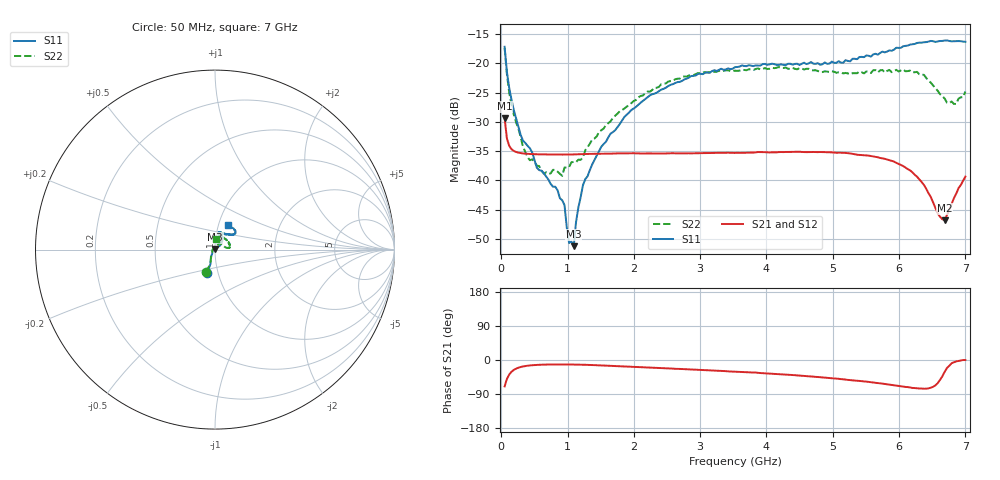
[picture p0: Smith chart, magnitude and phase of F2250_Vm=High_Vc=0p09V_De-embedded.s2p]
! Integrated Device Technology
! Corporate Headquarters
! 6024 Silver Creek Valley Road
! San Jose, CA 95138  USA
! Phone:  1-408-284-8200
! Toll Free:  1-800-223-1366
! Webpage:  http://www.idt.com/
! Timing and RF Division
! 515 Groton Road, Suite 102
! Westford, MA 01886-6024
! Device:  F2250
! Description: Voltage Variable RF Attenuator
! Frequency:  50.0 -  6000.00 MHz
! Package:  3x3 mm Thin QFN Plastic Package: 16 pin
! Ports:  2 RF, 3 DC
!  Pin  1  = GND
!  Pin  2  = NC
!  Pin  3  = RF1  = Port 1
!  Pin  4  = NC
!  Pin  5  = GND
!  Pin  6  = GND
!  Pin  7  = GND
!  Pin  8  = GND
!  Pin  9  = NC
!  Pin 10  = RF2  = Port 2
!  Pin 11  = NC
!  Pin 12  = GND
!  Pin 13  = GND
!  Pin 14  = VCNTRL
!  Pin 15  = VDD
!  Pin 16  = VMODE
! Vcntrl:  0.090 Volts
! Vmode:  +3.300 Volts
! Vdd:  +3.30  Volts
! Current:  1.245 mA
! Data:  The device was measured on a the F2250 evaluation board which has
!  individual transmission lines to the RF pins.  Data was collected
!  using a calibrated network analyzer.  The evaluation board was
!  de-embedded using a TRL calibration technique.
!  The reference plane is the edge of the package pin.
! Misc:  SN 10
!  Action Tracker AT0258
! Date Measured:  2014-11-26
! Date:  2015-10-15  MJV
! Note:
!  Integrated Device Technology supplies this data as a sample of measured
!  data at the package pin for this product.  Your particular data for this
!  product may vary.
!  Data was taken at 25 degrees C.
!  Integrated Device Technology reserves the right to change this data at anytime.
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# GHz S dB R 50
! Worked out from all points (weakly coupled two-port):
!   201 points, 50 MHz to 7 GHz, reference 50 ohm
!   highest |S21| = -29.38 dB at 50 MHz (marker M1); lowest = -46.8 dB at 6.687 GHz (marker M2)
!   lowest |S11| = -51.3 dB at 1.093 GHz (marker M3), VSWR 1.01, Z = 50 + j0.274 ohm
!   |S11| at or under -10 dB: start of sweep to end of sweep
!   |S22| runs from -39.2 to -17.4 dB; largest |S21 - S12| = 6.4e-05
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0.05  -17.18 -108.5  -29.38 -69.5  -29.38 -69.5  -17.37 -110.6
0.08475  -21.47 -107.4  -32.86 -50.1  -32.86 -50.1  -21.87 -109.0
0.15425  -26.23 -116.6  -34.68 -31.0  -34.68 -31.0  -27.10 -120.7
0.29325  -32.28 -127.5  -35.35 -18.5  -35.35 -18.4  -32.66 -133.5
0.3975  -34.11 -142.2  -35.48 -15.0  -35.48 -15.0  -36.08 -158.3
0.5365  -37.86 -154.5  -35.55 -12.9  -35.55 -12.9  -37.48 -180.0
0.64075  -38.76 -162.6  -35.58 -12.2  -35.58 -12.2  -38.88 160.6
0.91875  -43.41 156.3  -35.60 -11.8  -35.60 -11.8  -39.24 127.9
0.9535  -44.23 170.9  -35.60 -11.8  -35.60 -11.8  -37.79 124.2
1.023  -50.72 140.4  -35.59 -11.9  -35.59 -11.9  -37.73 108.0
1.0925  -51.26 90.1  -35.57 -12.0  -35.57 -12.0  -36.85 98.8
1.12725  -47.14 61.5  -35.56 -12.1  -35.56 -12.1  -36.91 91.6
1.2315  -40.84 40.8  -35.52 -12.5  -35.53 -12.5  -36.06 77.2
1.6485  -32.02 41.2  -35.44 -15.2  -35.44 -15.2  -29.91 59.9
2.37825  -24.76 46.7  -35.40 -21.0  -35.40 -21.0  -24.02 53.9
3.525  -20.65 71.7  -35.32 -30.6  -35.32 -30.6  -21.26 72.9
4.7065  -20.06 72.0  -35.16 -43.9  -35.16 -43.9  -21.21 70.4
5.85325  -17.79 40.5  -36.58 -64.8  -36.58 -64.9  -21.13 23.3
6.27025  -16.53 39.4  -39.39 -74.5  -39.40 -74.5  -21.46 8.6
6.68725  -16.11 47.8  -46.82 -31.2  -46.78 -30.7  -26.02 28.4
6.861  -16.22 54.5  -42.30 -3.7  -42.27 -3.7  -26.96 57.4
7  -16.32 62.4  -39.36 -0.1  -39.32 -0.3  -24.81 83.6
